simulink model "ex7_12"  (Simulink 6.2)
settings: Solver=ode5  SolverMode=SingleTasking  StartTime=0.0  StopTime=50  FixedStep=0.05  MaxStep=10  RelTol=1e-3  AbsTol=1e-6

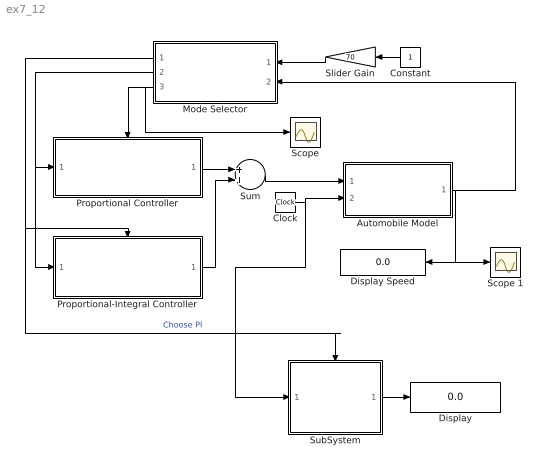
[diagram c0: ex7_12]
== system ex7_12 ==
  Automobile Model : Subsystem
  Clock : Clock
  Constant : Constant  Orientation=left
  Display : Display
  Display Speed : Display
  Mode Selector : Subsystem  Orientation=left
  Proportional Controller : Subsystem
  Proportional-Integral Controller : Subsystem
  Scope : Scope
  Scope 1 : Scope
  Slider Gain : Gain  Orientation=left  LoadFcn=slideg Load  Gain=70  mask(Slider Gain){}
  SubSystem : Subsystem
  Sum : Sum
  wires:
  Mode Selector/3(Choose P) -> Scope/1, Proportional Controller/Enable
  Proportional Controller/1(Commanded Thrust) -> Sum/1
  Proportional-Integral Controller/1(Commanded Thrust) -> Sum/2
  Sum/1 -> Automobile Model/1(Commanded Thrust)
  Mode Selector/2(Speed Error) -> Proportional Controller/1(Speed Error), Proportional-Integral Controller/1(Speed Error)
  Constant/1 -> Slider Gain/1
  Slider Gain/1 -> Mode Selector/1(Desired Speed)
  Automobile Model/1(Speed Out) -> Mode Selector/2(Actual  Speed), Scope 1/1, Display Speed/1
  Clock/1 -> Automobile Model/2(Time In), SubSystem/1(In1)
  Mode Selector/1(Choose PI) -> Proportional-Integral Controller/Enable, SubSystem/Trigger  "Choose PI"
  SubSystem/1(Out1) -> Display/1

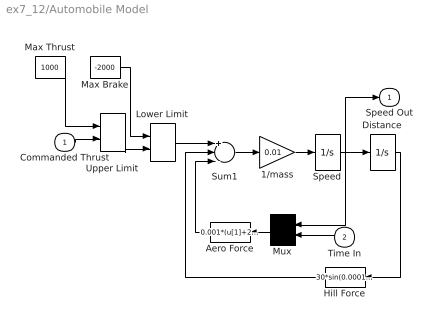
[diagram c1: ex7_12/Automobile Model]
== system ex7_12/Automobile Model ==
  Commanded Thrust : Inport  Port=1  LatchInput=off
  Time In : Inport  Orientation=left  Port=2  LatchInput=off
  1/mass : Gain  Gain=0.01
  Aero Force : Fcn  Orientation=left  Expr=0.001*(u[1]+20*sin(0.01*u[2]))^2
  Distance : Integrator
  Hill Force : Fcn  Orientation=left  Expr=30*sin(0.0001*u[1])
  Lower Limit : MinMax  Function=max  Inputs=2
  Max Brake : Constant  Value=-2000
  Max Thrust : Constant  Value=1000
  Mux : Mux  Orientation=left  Inputs=2
  Speed : Integrator
  Sum1 : Sum  Inputs=+--
  Upper Limit : MinMax  Inputs=2
  Speed Out : Outport  InitialOutput=0
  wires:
  Time In/1 -> Mux/2
  Lower Limit/1 -> Sum1/1
  Max Brake/1 -> Lower Limit/1
  Max Thrust/1 -> Upper Limit/1
  Upper Limit/1 -> Lower Limit/2
  1/mass/1 -> Speed/1
  Sum1/1 -> 1/mass/1
  Distance/1 -> Hill Force/1
  Hill Force/1 -> Sum1/2
  Aero Force/1 -> Sum1/3
  Speed/1 -> Mux/1, Speed Out/1, Distance/1
  Mux/1 -> Aero Force/1
  Commanded Thrust/1 -> Upper Limit/2

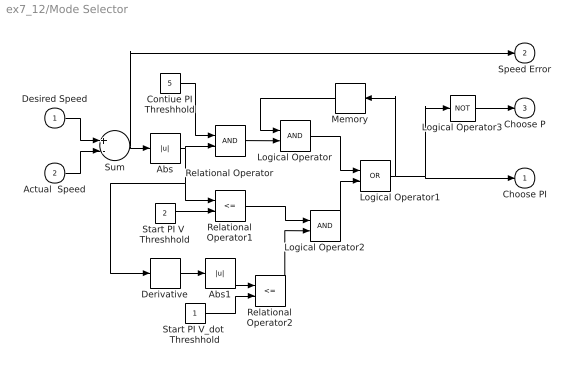
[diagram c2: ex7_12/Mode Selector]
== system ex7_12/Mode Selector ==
  Desired Speed : Inport  Port=1  LatchInput=off
  Actual  Speed : Inport  Port=2  LatchInput=off
  Abs : Abs
  Abs1 : Abs
  Contiue PI Threshhold : Constant  Value=5
  Derivative : Derivative
  Logical Operator : Logic
  Logical Operator1 : Logic  Operator=OR
  Logical Operator2 : Logic
  Logical Operator3 : Logic  Operator=NOT  Inputs=1
  Memory : Memory  Orientation=left
  Relational Operator : RelationalOperator
  Relational Operator1 : RelationalOperator  Operator=<=
  Relational Operator2 : RelationalOperator  Operator=<=
  Start PI V  Threshhold : Constant  Value=2
  Start PI V_dot  Threshhold : Constant
  Sum : Sum  Inputs=+-
  Choose PI : Outport  InitialOutput=0
  Speed Error : Outport  Port=2  InitialOutput=0
  Choose P : Outport  Port=3  InitialOutput=0
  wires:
  Desired Speed/1 -> Sum/1
  Actual  Speed/1 -> Sum/2
  Contiue PI Threshhold/1 -> Relational Operator/1
  Abs/1 -> Relational Operator/2, Relational Operator1/1, Derivative/1
  Start PI V  Threshhold/1 -> Relational Operator1/2
  Start PI V_dot  Threshhold/1 -> Relational Operator2/2
  Abs1/1 -> Relational Operator2/1
  Relational Operator/1 -> Logical Operator/2
  Logical Operator/1 -> Logical Operator1/1
  Relational Operator1/1 -> Logical Operator2/1
  Relational Operator2/1 -> Logical Operator2/2
  Logical Operator2/1 -> Logical Operator1/2
  Memory/1 -> Logical Operator/1
  Logical Operator1/1 -> Memory/1, Choose PI/1, Logical Operator3/1
  Sum/1 -> Abs/1, Speed Error/1
  Derivative/1 -> Abs1/1
  Logical Operator3/1 -> Choose P/1

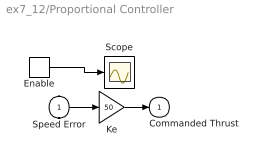
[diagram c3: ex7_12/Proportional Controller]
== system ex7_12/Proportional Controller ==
  Speed Error : Inport  Port=1  LatchInput=off
  Enable : EnablePort  StatesWhenEnabling=reset  ShowOutputPort=on
  Ke : Gain  Gain=50
  Scope : Scope
  Commanded Thrust : Outport  OutputWhenDisabled=reset  InitialOutput=0
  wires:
  Speed Error/1 -> Ke/1
  Ke/1 -> Commanded Thrust/1
  Enable/1 -> Scope/1

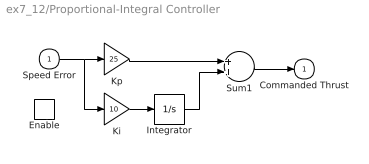
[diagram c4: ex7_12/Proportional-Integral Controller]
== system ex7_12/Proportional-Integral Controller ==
  Speed Error : Inport  Port=1  LatchInput=off
  Enable : EnablePort  StatesWhenEnabling=reset
  Integrator : Integrator
  Ki : Gain  Gain=10
  Kp : Gain  Gain=25
  Sum1 : Sum
  Commanded Thrust : Outport  OutputWhenDisabled=reset  InitialOutput=0
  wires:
  Ki/1 -> Integrator/1
  Speed Error/1 -> Kp/1, Ki/1
  Kp/1 -> Sum1/1
  Integrator/1 -> Sum1/2
  Sum1/1 -> Commanded Thrust/1

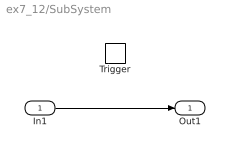
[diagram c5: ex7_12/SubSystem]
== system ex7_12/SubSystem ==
  In1 : Inport  Port=1  LatchInput=off
  Trigger : TriggerPort
  Out1 : Outport
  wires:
  In1/1 -> Out1/1
